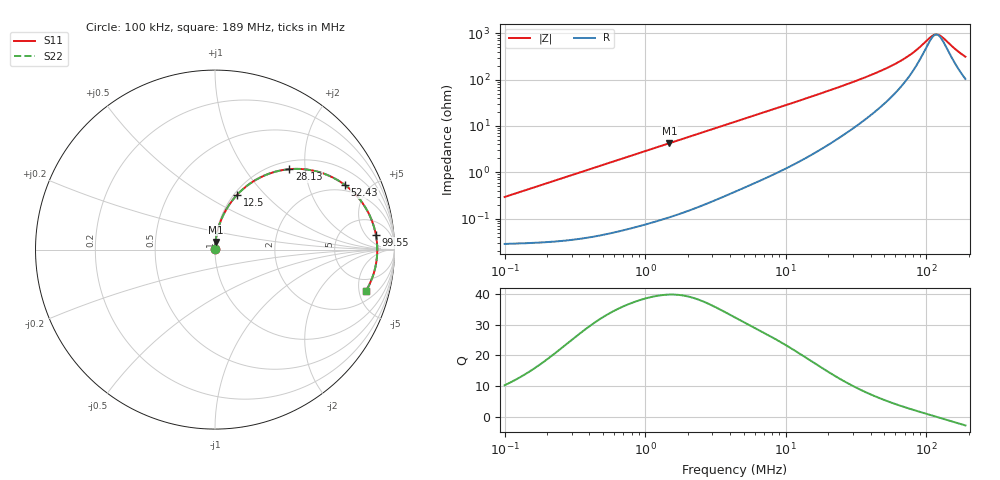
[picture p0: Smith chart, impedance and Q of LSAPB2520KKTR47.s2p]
! LSAPB2520KKTR47  S-PARAMETER MODEL  ( General Type )
! Model Generated by TAIYO YUDEN Corporation (http://www.ty-top.com)
! Version 3.0
! TAIYO YUDEN Control No. 20210629
! Copyright(c) 2015 TAIYO YUDEN CO.,LTD. All Rights Reserved.
! Product Description (link to TY-COMPAS)
! https://ds.yuden.co.jp/TYCOMPAS/or/detail?pn=LSAPB2520KKTR47M&u=M
! Products Name : Inductors
! Characteristics :
!  Inductance : 0.47 uH , SRF(min) : -Hz , DC Resistance(max) : 0.029 Ohm
!  Rated Current : Saturation :5700 mA , Temp Rise : 4000 mA (40 degC)
!  Case Size : 2.5 x 2.0 / 0.098 x 0.079 [mm/inch] , Thickness : 1 / 0.039 [mm/inch]
!  (Conditions: Temperature = 25 degC , DC Bias Current/Voltage = 0A / 0V)
! External Node Assignments :
!  1  o---GGG---o  2
! GND o---------o GND
! Frequency Range : 0.1MHz  -  189.042664MHz  [ 402 STEP ]
# MHz S RI R 50
! Freq[MHz].  S11 Real  S11 Imag  S21 Real  S21 Imag  S12 Real  S12 Imag  S22 Real  S22 Imag
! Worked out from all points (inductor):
!   401 points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, 100 kHz to 189 MHz, reference 50 ohm
!   read as one part in series: L = 463 nH near 103.8 kHz
!   highest Q = 39.8 at 1.484 MHz (marker M1), where L = 455 nH
!   self-resonance near 117.5 MHz
!   S11 on the Smith chart (normalised r, x): 100 kHz: 1.00, +0.01; 12.5 MHz: 1.03, +0.70; 28.13 MHz: 1.15, +1.65; 52.43 MHz: 1.69, +3.51; 99.55 MHz: 11, +9; 189 MHz: 3.07, -5.90
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0.1  0.000293 0.00291  0.9997 -0.00291  0.9997 -0.00291  0.000293 0.00291
0.353854  0.000476 0.0102  0.9995 -0.0102  0.9995 -0.0102  0.000476 0.0102
1.252125  0.00219 0.0357  0.9978 -0.0357  0.9978 -0.0357  0.00219 0.0357
1.483782  0.00285 0.0423  0.9971 -0.0423  0.9971 -0.0423  0.00285 0.0423
4.347904  0.0185 0.1202  0.9815 -0.1202  0.9815 -0.1202  0.0185 0.1202
7.950688  0.055 0.2095  0.945 -0.2095  0.945 -0.2095  0.055 0.2095
12.50254  0.1221 0.3041  0.8779 -0.3041  0.8779 -0.3041  0.1221 0.3041
15.38522  0.173 0.3514  0.827 -0.3514  0.827 -0.3514  0.173 0.3514
20.41619  0.269 0.41  0.731 -0.41  0.731 -0.41  0.269 0.41
28.1338  0.4141 0.448  0.5859 -0.448  0.5859 -0.448  0.4141 0.448
38.04441  0.5701 0.4346  0.4299 -0.4346  0.4299 -0.4346  0.5701 0.4346
52.42575  0.7246 0.3594  0.2754 -0.3594  0.2754 -0.3594  0.7246 0.3594
54.44117  0.7405 0.3468  0.2595 -0.3468  0.2595 -0.3468  0.7405 0.3468
75.02072  0.8479 0.2176  0.1521 -0.2176  0.1521 -0.2176  0.8479 0.2176
85.60932  0.8761 0.1562  0.1239 -0.1562  0.1239 -0.1562  0.8761 0.1562
99.55252  0.8964 0.0827  0.1036 -0.0827  0.1036 -0.0827  0.8964 0.0827
111.4809  0.9034 0.0265  0.0966 -0.0265  0.0966 -0.0265  0.9034 0.0265
117.9709  0.9042 -0.00183  0.0958 0.00183  0.0958 0.00183  0.9042 -0.00183
122.5061  0.9038 -0.0207  0.0962 0.0207  0.0962 0.0207  0.9038 -0.0207
132.1062  0.9005 -0.0583  0.0995 0.0583  0.0995 0.0583  0.9005 -0.0583
165.6609  0.8717 -0.1688  0.1283 0.1688  0.1283 0.1688  0.8717 -0.1688
189.0427  0.8417 -0.2297  0.1583 0.2297  0.1583 0.2297  0.8417 -0.2297
